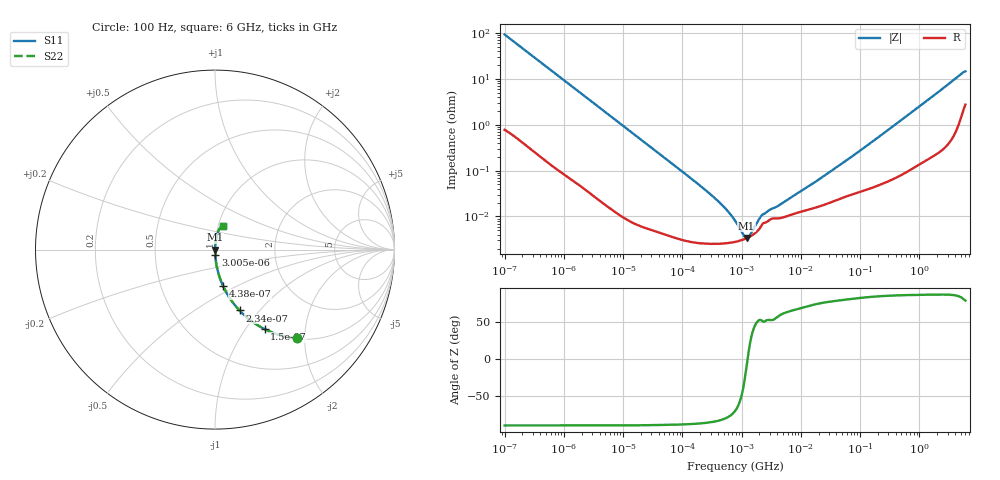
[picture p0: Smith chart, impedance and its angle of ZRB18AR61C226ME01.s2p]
!Murata Part Number: ZRB18AR61C226ME01
!These Parameters are Measured in Series Mode Connection
!Data Generated on Jun 10, 2025
!  o--ll--o
!Port1  Port2
!  o------o
!Operation Temp=25[degC], DC Bias Voltage=0[V]
!Freq. Start=100[Hz] Stop=6[GHz] 401[Steps]
# Hz S RI R 50
!Freq.(Hz) S11(Real) S11(Imag) S21(Real) S21(Imag) S12(Real) S12(Imag) S22(Real) S22(Imag)
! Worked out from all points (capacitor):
!   401 points, 100 Hz to 6 GHz, reference 50 ohm
!   read as one part in series: C = 17.3 uF near 109 Hz
!   lowest |Z| = 3.41 mohm at 1.212 MHz (marker M1)
!   series resonance near 1.263 MHz, so ESL is about 920 pH
!   S11 on the Smith chart (normalised r, x): 100 Hz: 1.02, -1.83; 150 Hz: 1.01, -1.23; 234 Hz: 1.01, -0.79; 438 Hz: 1.00, -0.42; 3.005 kHz: 1.00, -0.06; 6 GHz: 1.05, +0.28
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100  0.4574 -0.494  0.5426 0.494  0.5426 0.494  0.4574 -0.494
150  0.2761 -0.4427  0.7239 0.4427  0.7239 0.4427  0.2761 -0.4427
234  0.1366 -0.3391  0.8634 0.3391  0.8634 0.3391  0.1366 -0.3391
438  0.0443 -0.2015  0.9557 0.2015  0.9557 0.2015  0.0443 -0.2015
897  0.0115 -0.1023  0.9885 0.1023  0.9885 0.1023  0.0115 -0.1023
2008  0.00259 -0.0463  0.9974 0.0463  0.9974 0.0463  0.00259 -0.0463
3005  0.00126 -0.0311  0.9987 0.0311  0.9987 0.0311  0.00126 -0.0311
40335  5.01e-05 -0.00235  0.9999 0.00235  0.9999 0.00235  5.01e-05 -0.00235
231233  2.58e-05 -0.0004  1 0.0004  1 0.0004  2.58e-05 -0.0004
413847  2.54e-05 -0.000206  1 0.000206  1 0.000206  2.54e-05 -0.000206
647581  2.68e-05 -0.000108  1 0.000108  1 0.000108  2.68e-05 -0.000108
774597  2.79e-05 -7.67e-05  1 7.67e-05  1 7.67e-05  2.79e-05 -7.67e-05
1212075  3.35e-05 -6.1e-06  1 6.1e-06  1 6.1e-06  3.35e-05 -6.1e-06
1896632  4.96e-05 6.27e-05  1 -6.27e-05  1 -6.27e-05  4.96e-05 6.27e-05
2169299  6.34e-05 8.26e-05  0.9999 -8.26e-05  0.9999 -8.26e-05  6.34e-05 8.26e-05
4246196  9.11e-05 0.000148  0.9999 -0.000148  0.9999 -0.000148  9.11e-05 0.000148
1.555665e7  0.000149 0.000488  0.9999 -0.000488  0.9999 -0.000488  0.000149 0.000488
7.455971e7  0.000307 0.00204  0.9997 -0.00204  0.9997 -0.00204  0.000307 0.00204
3.124326e8  0.00066 0.008  0.9993 -0.008  0.9993 -0.008  0.00066 0.008
1.712697e9  0.00378 0.0417  0.9962 -0.0417  0.9962 -0.0417  0.00378 0.0417
4.796499e9  0.0249 0.1152  0.9751 -0.1152  0.9751 -0.1152  0.0249 0.1152
6e9  0.0447 0.1318  0.9553 -0.1318  0.9553 -0.1318  0.0447 0.1318
